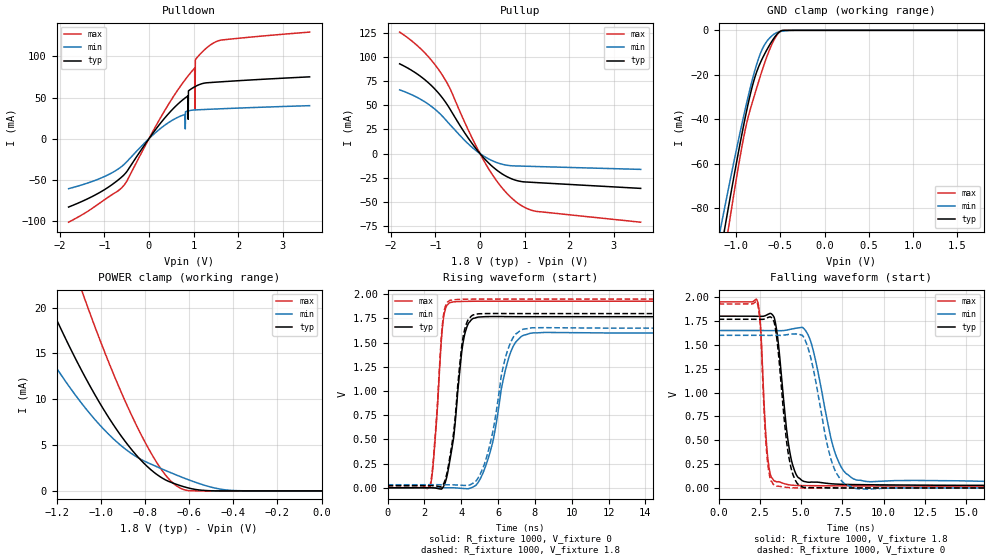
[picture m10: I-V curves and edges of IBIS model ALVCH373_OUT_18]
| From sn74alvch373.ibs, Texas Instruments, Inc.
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[Model]   ALVCH373_OUT_18
Model_type  3-state
Enable   Active-Low
Vref =   0
Rref =   1000
Cref =   30p
Vmeas =   0.9
| variable   typ   min   max
C_comp   7.02pF   6.18pF   7.76pF
| C_pullup   8.70pF   6.86pF   9.47pF
| C_pulldown   16.90pF   7.22pF   54.41pF
| C_tri-state   7.02pF   6.18pF   7.76pF
[Temperature Range]   40   100   -40
| Ambient temperature   25   85   -40
[Voltage range]   1.8   1.65   1.95
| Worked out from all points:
|   slope of the pulldown table from 0 to 0.27 V, typ, clamps not added: 13.8 ohm
|   slope of the pullup table from 0 to 0.27 V, typ, clamps not added: 20.7 ohm
|   GND clamp passes 1 mA (typ) near -0.52 V on its own axis
|   POWER clamp passes 1 mA (typ) near -0.69 V on its own axis
|   rising waveform, R_fixture 1000, V_fixture 0: 20-80 % time 586ps typ, 995ps min, 391ps max; typ from 0 V to 1.77 V
|   falling waveform, R_fixture 1000, V_fixture 1.8: 20-80 % time 651ps typ, 1.19ns min, 347ps max; typ from 1.8 V to 0.023 V
|   rising waveform, R_fixture 1000, V_fixture 1.8: 20-80 % time 583ps typ, 942ps min, 389ps max; typ from 0.023 V to 1.8 V
|   falling waveform, R_fixture 1000, V_fixture 0: 20-80 % time 607ps typ, 1.08ns min, 331ps max; typ from 1.77 V to 0 V
[GND Clamp]
| ALVCH373_OUT_18
|   Voltage   I(typ)   I(min)   I(max)
-1.8V     -251.5mA   -223mA     -282.5mA
-1.18V    -100.5mA   -89.65mA   -112.8mA
-1.135V   -90.14mA   -80.51mA   -101mA
-1.11V    -84.43mA   -75.49mA   -94.56mA
-1.09V    -79.91mA   -71.51mA   -89.44mA
-1.07V    -75.42mA   -67.55mA   -84.36mA
-915mV    -42.39mA   -38.3mA    -47.91mA
-815mV    -24.67mA   -21.69mA   -31.96mA
-700mV    -12.26mA   -7.984mA   -17.13mA
-565mV    -3.023mA   -1.514mA   -3.748mA
-475mV    -42.56uA   -359uA     -30.01uA
1.8V      72.12pA    23.02nA    9.218pA
[POWER Clamp]
| ALVCH373_OUT_18
|   Voltage   I(typ)   I(min)   I(max)
-1.8V     57mA       41.48mA    82.63mA
-1.39V    29.42mA    21.07mA    45.16mA
-1.25V    21.36mA    15.28mA    33.85mA
-1.085V   13.07mA    9.514mA    21.81mA
-1.07V    12.39mA    9.055mA    20.79mA
-960mV    7.858mA    6.084mA    13.8mA
-865mV    4.653mA    4.149mA    8.505mA
-760mV    2.053mA    2.789mA    3.63mA
-670mV    829.8uA    1.861mA    798.1uA
-610mV    364.7uA    1.286mA    56uA
-440mV    2.059uA    132.1uA    46.48nA
-16.28fV  72.12pA    575pA      10.31pA
[Pulldown]
| ALVCH373_OUT_18
|   Voltage   I(typ)   I(min)   I(max)
-1.8V     -82.99mA   -60.68mA   -101.4mA
-565mV    -44.24mA   -31.63mA   -56.91mA
710mV     45.04mA    27.51mA    64.13mA
875mV     52.01mA    33.72mA    76.14mA
880mV     23.63mA    33.79mA    76.48mA
885mV     58.02mA    33.85mA    76.82mA
1.02V     62.91mA    34.93mA    85.51mA
1.025V    63.06mA    34.95mA    85.74mA
1.03V     63.21mA    34.96mA    34.89mA
1.04V     63.5mA     34.99mA    95.36mA
1.33V     68.06mA    35.71mA    112mA
3.6V      75.16mA    40.15mA    129.5mA
[Pullup]
| ALVCH373_OUT_18
|   Voltage   I(typ)   I(min)   I(max)
-1.8V     93.1mA     66.08mA    126mA
-1.305V   79.16mA    55.62mA    107.7mA
-1.09V    70.61mA    48.99mA    96.92mA
-900mV    61.14mA    41.46mA    85.33mA
-680mV    46.8mA     30.45mA    68.18mA
-250mV    15.23mA    9.524mA    23.26mA
130mV     -6.768mA   -3.901mA   -10.86mA
465mV     -20.13mA   -10.67mA   -33.86mA
805mV     -27.75mA   -12.84mA   -49.92mA
1.03V     -29.51mA   -13.14mA   -56.52mA
1.26V     -30.1mA    -13.44mA   -59.95mA
3.6V      -36.12mA   -16.42mA   -71.2mA
[Ramp]
| ALVCH373_OUT_18
| variable   typ   min   max
dV/dt_r   1.07/6.02E-10   0.97/1.05E-09   1.16/3.99E-10
dV/dt_f   1.08/6.67E-10   0.99/1.25E-09   1.18/3.54E-10
R_load = 1000
[Rising Waveform]
| ALVCH373_OUT_18
R_fixture =   1000
C_fixture =   0
L_fixture =   0
V_fixture =   0
V_fixture_min = 0
V_fixture_max = 0
|   Time   V(typ)   V(min)   V(max)
0s        45.86pV    4.067nV    33.01pV
2.33ns    181.5uV    369.9uV    21.9mV
3ns       846.6uV    87.25uV    1.692V
3.4ns     299.8mV    -146.4uV   1.914V
4.035ns   1.415V     -6.208mV   1.926V
4.385ns   1.697V     -9.586mV   1.927V
5.465ns   1.769V     302.1mV    1.928V
6.72ns    1.768V     1.418V     1.928V
7.745ns   1.768V     1.596V     1.928V
40ns      1.768V     1.6V       1.928V
[Falling Waveform]
| ALVCH373_OUT_18
R_fixture =   1000
C_fixture =   0
L_fixture =   0
V_fixture =   1.8
V_fixture_min = 1.65
V_fixture_max = 1.95
|   Time   V(typ)   V(min)   V(max)
0s        1.8V       1.65V      1.95V
2.365ns   1.799V     1.65V      1.951V
2.545ns   1.798V     1.65V      1.689V
2.975ns   1.818V     1.649V     320.9mV
3.5ns     1.671V     1.649V     65.7mV
4.33ns    360.2mV    1.662V     31.59mV
5.185ns   67.48mV    1.667V     24.83mV
7.07ns    41.41mV    360mV      22.47mV
8.33ns    35.35mV    84.89mV    21.61mV
40ns      23.36mV    36.89mV    18.99mV
[Rising Waveform]
| ALVCH373_OUT_18
R_fixture =   1000
C_fixture =   0
L_fixture =   0
V_fixture =   1.8
V_fixture_min = 1.65
V_fixture_max = 1.95
|   Time   V(typ)   V(min)   V(max)
0s        23.08mV    31.17mV    18.98mV
2.33ns    23.05mV    31.47mV    42.07mV
2.995ns   24.69mV    30.86mV    1.717V
3.405ns   344mV      30.55mV    1.938V
4.03ns    1.466V     25.35mV    1.948V
4.36ns    1.732V     22.91mV    1.949V
5.26ns    1.8V       244.9mV    1.95V
6.445ns   1.8V       1.375V     1.95V
7.395ns   1.8V       1.64V      1.95V
40ns      1.8V       1.65V      1.95V
[Falling Waveform]
| ALVCH373_OUT_18
R_fixture =   1000
C_fixture =   0
L_fixture =   0
V_fixture =   0
V_fixture_min = 0
V_fixture_max = 0
|   Time   V(typ)   V(min)   V(max)
0s        1.768V     1.6V       1.928V
2.355ns   1.767V     1.6V       1.93V
2.545ns   1.766V     1.6V       1.643V
2.96ns    1.784V     1.599V     281.4mV
3.49ns    1.613V     1.6V       19.86mV
4.26ns    318.5mV    1.609V     4.04mV
5.15ns    6.702mV    1.58V      313.8uV
6.89ns    924.5uV    255.8mV    225.5uV
8.26ns    268uV      -3.162mV   224.7uV
40ns      20.44uV    113.4uV    1.433uV
